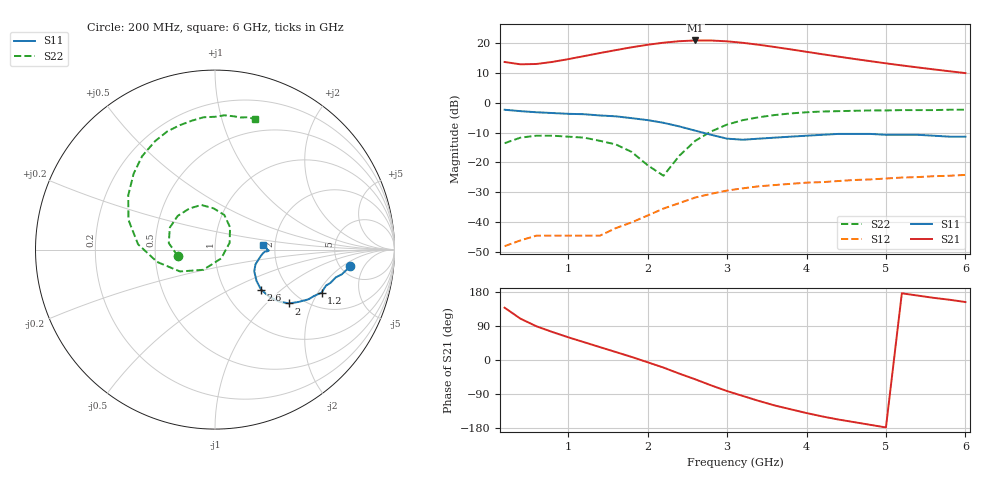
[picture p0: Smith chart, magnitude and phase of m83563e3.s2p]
!	MGA-83563 S PARAMETERS
!	Vd = 3 V L=1.2 nH  LAST UPDATED 10-15-97
# ghz	s ma r	50
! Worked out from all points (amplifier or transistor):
!   30 points, 200 MHz to 6 GHz, reference 50 ohm
!   highest |S21| = 20.8 dB at 2.6 GHz (marker M1)
!   |S21| within 3 dB of that: 1.646 GHz to 3.805 GHz (2.159 GHz wide, 79.2 % of centre)
!   unconditionally stable (mu >= 1): start of sweep to end of sweep
!   at 1.2 GHz: K = 7.54, MAG = 18.2 dB, |S12| = -44.4 dB
!   at 3.2 GHz: K = 1.24, MAG = 21.3 dB, |S12| = -28.6 dB
!   at 6 GHz: K = 1.18, MAG = 14.4 dB, |S12| = -24.2 dB
!   S11 on the Smith chart (normalised r, x): 200 MHz: 6.13, -2.69; 1.2 GHz: 2.65, -2.15; 2 GHz: 1.70, -1.38; 2.6 GHz: 1.47, -0.74; 6 GHz: 1.73, +0.11
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0.2  0.76 -7.0  4.77 138.0  0.004 57.0  0.21 -170.0
0.4  0.72 -11.0  4.36 109.0  0.005 43.0  0.26 172.0
0.6  0.69 -13.0  4.42 89.0  0.006 40.0  0.28 154.0
1  0.65 -18.0  5.32 60.0  0.006 50.0  0.27 122.0
1.2  0.64 -22.0  5.98 47.0  0.006 62.0  0.26 107.0
1.4  0.61 -25.0  6.73 34.0  0.006 76.0  0.23 92.0
1.6  0.59 -28.0  7.54 21.0  0.008 88.0  0.2 75.0
1.8  0.55 -32.0  8.4 8.0  0.01 96.0  0.15 56.0
2  0.51 -36.0  9.25 -6.0  0.013 100.0  0.09 25.0
2.2  0.46 -39.0  10.02 -20.0  0.017 100.0  0.06 -55.0
2.4  0.4 -41.0  10.61 -36.0  0.021 97.0  0.13 -120.0
2.6  0.34 -41.0  10.92 -51.0  0.026 93.0  0.23 -148.0
2.8  0.29 -37.0  10.9 -67.0  0.03 88.0  0.33 -168.0
3  0.25 -29.0  10.56 -82.0  0.034 82.0  0.43 176.0
3.2  0.24 -20.0  9.97 -95.0  0.037 76.0  0.51 161.0
3.4  0.25 -12.0  9.25 -108.0  0.04 71.0  0.57 148.0
3.6  0.26 -7.0  8.49 -120.0  0.042 67.0  0.62 137.0
4  0.28 -2.0  7.06 -140.0  0.046 59.0  0.69 119.0
4.2  0.29 -2.0  6.43 -149.0  0.047 56.0  0.71 112.0
4.6  0.3 -1.0  5.37 -164.0  0.051 51.0  0.73 100.0
5.2  0.29 0.0  4.18 176.0  0.056 44.0  0.75 86.0
6  0.27 6.0  3.11 153.0  0.062 35.0  0.76 73.0
